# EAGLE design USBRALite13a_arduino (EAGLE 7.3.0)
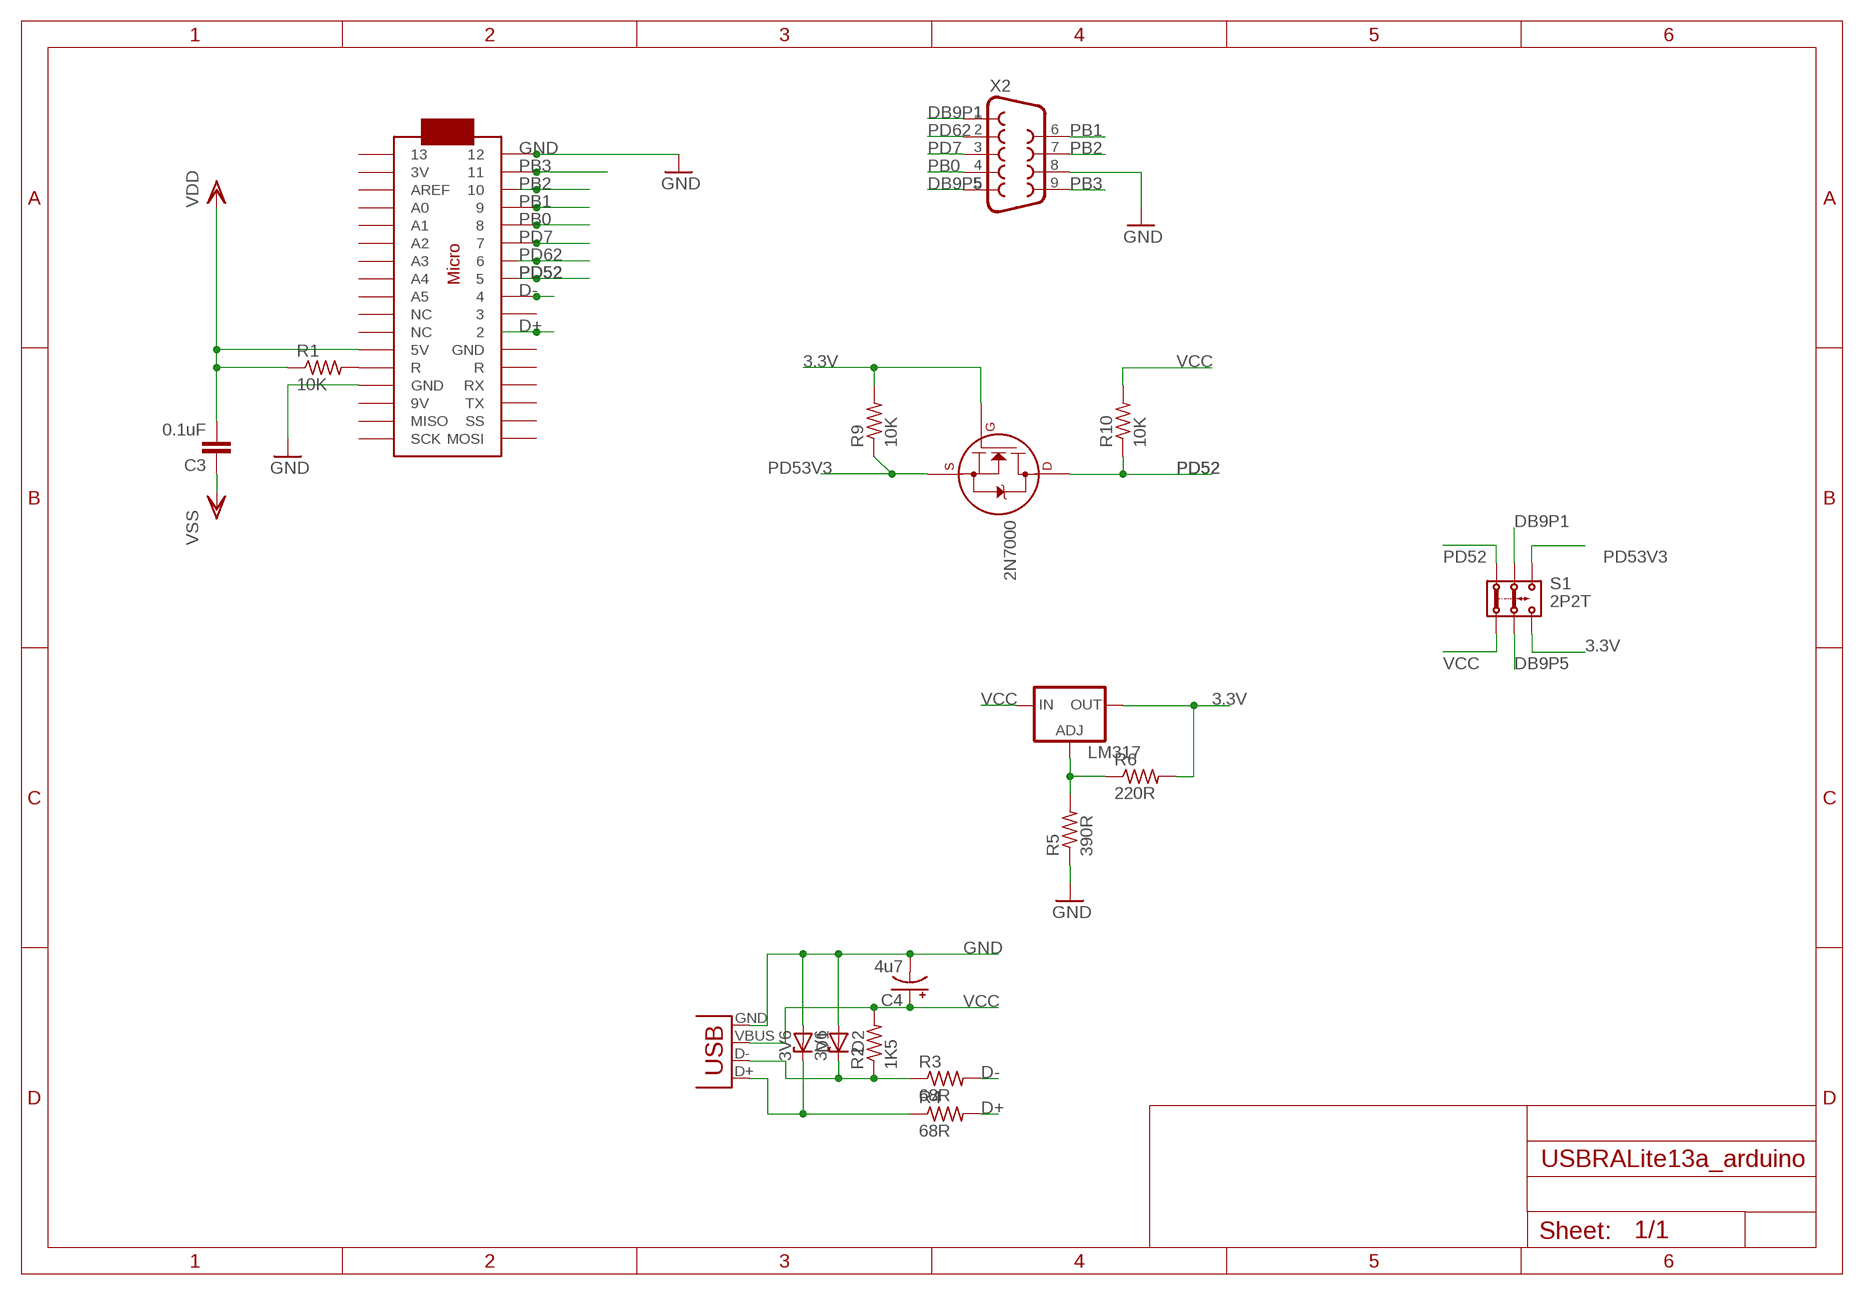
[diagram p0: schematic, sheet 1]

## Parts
2N7000  2N7000_TO92  [TO-92]
C3  0.1uF  C-EU050-024X044  [C050-024X044]
C4  4u7  CPOL-USE2.5-6  [E2,5-6]
D1  3V6  ZENER-DIODEZD-5  [ZDIO-5]
D2  3V6  ZENER-DIODEZD-5  [ZDIO-5]
LM317  LM317TS  [317TS]
R1  10K  R-US_0207/10  [0207/10]
R2  1K5  R-US_0207/10  [0207/10]
R3  68R  R-US_0207/10  [0207/10]
R4  68R  R-US_0207/10  [0207/10]
R5  390R  R-US_0207/10  [0207/10]
R6  220R  R-US_0207/10  [0207/10]
R9  10K  R-US_0207/10  [0207/10]
R10  10K  R-US_0207/10  [0207/10]
S1  2P2T  [2P2T]
U$2  ARDUINOMICRO  [ARDUINOMICRO]
X1  USBPTH  [USB-B-PTH]
X2  DB9MALE  [DB9_MALE]

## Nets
3.3V: 2N7000.2(G) LM317.2(OUT) R6.2 R9.2 S1.3.2
D+: R4.2 U$2.P$11
D-: R3.2 U$2.P$9
DB9P1: S1.2.1 X2.1
DB9P5: S1.2.2 X2.5
GND: C3.1 C4.- D1.A D2.A R5.1 U$2.P$1 U$2.P$12(GND) X1.GND X2.8 ; supply symbol labelled VSS
N$1: R1.2 U$2.P$13(R)
N$5: LM317.1(ADJ) R5.2 R6.1
N$8: D1.C R4.1 X1.D+
N$9: D2.C R2.1 R3.1 X1.D-
PB0: U$2.P$5 X2.4
PB1: U$2.P$4 X2.6
PB2: U$2.P$3 X2.7
PB3: U$2.P$2 X2.9
PD7: U$2.P$6 X2.3
PD52: 2N7000.3(D) R10.1 S1.1.1 U$2.P$8
PD53V3: 2N7000.1(S) R9.1 S1.3.1
PD62: U$2.P$7 X2.2
VCC: C3.2 C4.+ LM317.3(IN) R1.1 R2.2 R10.2 S1.1.2 U$2.P$23(5V) X1.VBUS ; supply symbol labelled VDD
Unconnected: U$2.P$10 U$2.P$14(RX) U$2.P$15(TX) U$2.P$16(SS) U$2.P$17(MOSI) U$2.P$18(SCK) U$2.P$19(MISO) U$2.P$20(9V) U$2.P$21(GND) U$2.P$22(R) U$2.P$24(NC) U$2.P$25(NC) U$2.P$26(A5) U$2.P$27(A4) U$2.P$28(A3) U$2.P$29(A2) U$2.P$30(A1) U$2.P$31(A0) U$2.P$32(AREF) U$2.P$33(3V) U$2.P$34

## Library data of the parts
2N7000 = transistors:2N700*: 2N7000, 2N7002, NDS7002A N-channel enhancement mode MOSFET
C3 = rcl:C-EU: CAPACITOR, European symbol
C4 = adafruit:CPOL-US: POLARIZED CAPACITOR, American symbol
D1 D2 = diode:ZENER-DIODE: Z-Diode
LM317 = v-reg:LM317TS: VOLTAGE REGULATOR
R1-R6 R9 R10 = adafruit:R-US_: RESISTOR, American symbol
S1 = Itead_BP_110825:2P2T: BAS011
U$2 = adafruit:ARDUINOMICRO
X1 = SparkFun:USB: USB Connectors USB-B-PTH is fully proven SKU : PRT-00139 USB-miniB is fully proven SKU : PRT-00587 USB-A-PCB is untested. USB-A-H is throughly reviewed, but untested. Spark Fun Electronics SKU : PRT-00437 USB-B-SMT is throughly reviewed, but untested. Needs silkscreen touching up. USB-A-S has not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
X2 = SparkFun:DB9: DB9 Connector Standard DB9 (D-Sub 9) serial connector. Can be used for CAN bus as well as RS485 and RS232. Footprint production proven. Spark Fun Electronics SKU : PRT-00429

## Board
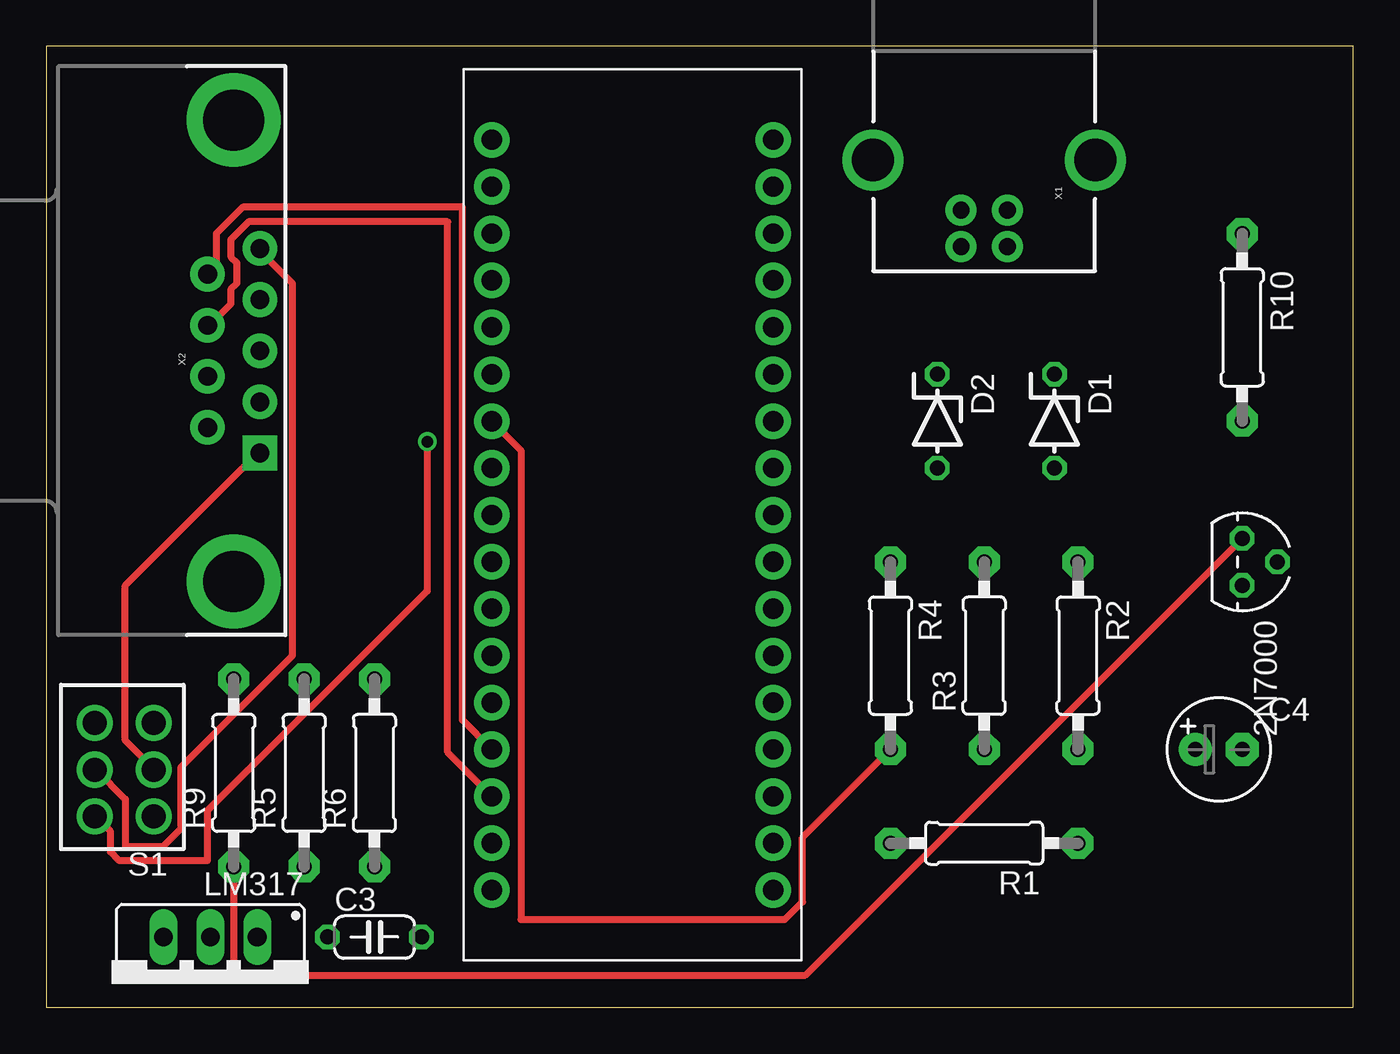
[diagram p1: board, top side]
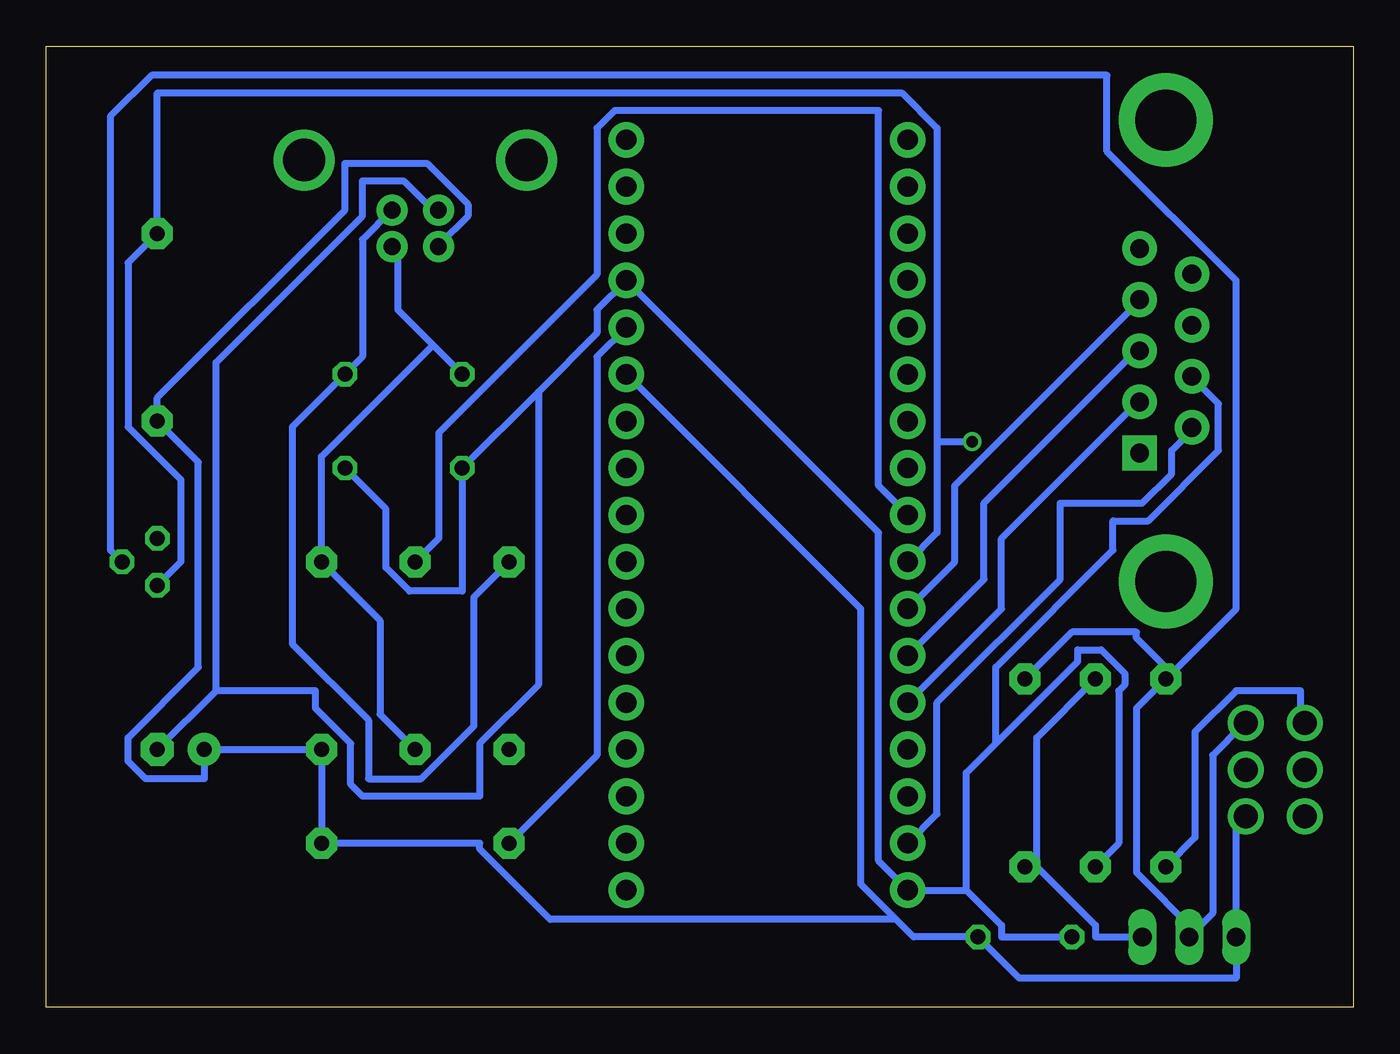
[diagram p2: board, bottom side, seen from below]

Size 70.79 x 52.06 mm. Coordinates in mm from the lower left corner, seen from the top.
Outline: 0,0 70.79,0 70.79,52.06 0,52.06 0,0
Copper layers (1*16): Top 0.035mm / dielectric 1.5mm / Bottom 0.035mm
Design rules "default *": minimum track width 15mil, minimum drill 24mil, track to track 12mil, track to pad 12mil, pad to pad 12mil, via to via 12mil, smd to smd 12mil, copper to edge 40mil, drill to drill 8mil, minimum pad ring 10mil, minimum via ring 8mil, stop-mask expansion 4mil, vias tented up to drill 0mil, thermal gap 10mil

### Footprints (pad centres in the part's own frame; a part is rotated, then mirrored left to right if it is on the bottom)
TO-92 = drill 0.813 octagon: 1 -1.27,0; 2 0,1.905; 3 1.27,0
C050-024X044 = drill 0.813 octagon: 1 -2.54,0; 2 2.54,0
E2,5-6 = drill 0.813 pad 1.778: + -1.27,0 | drill 0.813 pad 1.778 octagon: - 1.27,0
ZDIO-5 = drill 0.813 octagon: A 2.54,0; C -2.54,0
317TS = drill 1.016 long: 1 -2.54,-2.54; 2 0,-2.54; 3 2.54,-2.54
0207/10 = drill 0.813 pad 1.676 octagon: 1 -5.08,0; 2 5.08,0
2P2T = drill 1.3 pad 1.93: 1.1 -3.635,-0.085; 1.2 -3.635,-3.285; 2.1 -1.095,-0.085; 2.2 -1.095,-3.285; 3.1 1.445,-0.085; 3.2 1.445,-3.285
ARDUINOMICRO = drill 1.1 pad 1.93: P$1 -20.32,7.62; P$2 -17.78,7.62; P$3 -15.24,7.62; P$4 -12.7,7.62; P$5 -10.16,7.62; P$6 -7.62,7.62; P$7 -5.08,7.62; P$8 -2.54,7.62; P$9 0,7.62; P$10 2.54,7.62; P$11 5.08,7.62; P$12 12.7,-7.62; P$13 10.16,-7.62; P$14 12.7,7.62; P$15 15.24,7.62; P$16 17.78,7.62; P$17 20.32,7.62; P$18 20.32,-7.62; P$19 17.78,-7.62; P$20 15.24,-7.62; P$21 7.62,7.62; P$22 10.16,7.62; P$23 7.62,-7.62; P$24 5.08,-7.62; P$25 2.54,-7.62; P$26 0,-7.62; P$27 -2.54,-7.62; P$28 -5.08,-7.62; P$29 -7.62,-7.62; P$30 -10.16,-7.62; P$31 -12.7,-7.62; P$32 -15.24,-7.62; P$33 -17.78,-7.62; P$34 -20.32,-7.62
USB-B-PTH = drill 0.914 pad 1.676: D+ 0,1.25; D- 1.981,1.25; GND 0,-1.25; VBUS 1.981,-1.25 | drill 2.286: S1 -2.718,-6.02; S2 -2.718,6.02
DB9_MALE = drill 1.016 pad 1.88: 1 5.54,-1.42; 2 2.77,-1.42; 3 0,-1.42; 4 -2.77,-1.42; 6 4.15,1.42; 7 1.38,1.42; 8 -1.38,1.42; 9 -4.15,1.42 | drill 1.016 pad 1.88 square: 5 -5.54,-1.42 | drill 3.302 pad 5.08: G1 -12.5,0; G2 12.5,0

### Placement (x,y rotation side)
2N7000  64.77,24.13 270 top
C3  17.78,3.81 0 top
C4  63.5,13.97 0 top
D1  54.61,31.75 270 top
D2  48.26,31.75 270 top
LM317  8.89,1.27 180 top
R1  50.8,8.89 180 top
R2  55.88,19.05 270 top
R3  50.8,19.05 90 top
R4  45.72,19.05 270 top
R5  13.97,12.7 90 top
R6  17.78,12.7 90 top
R9  10.16,12.7 90 top
R10  64.77,36.83 270 top
S1  2.54,13.97 90 top
U$2  31.75,26.67 90 top
X1  50.8,43.18 270 top
X2  10.16,35.56 90 top

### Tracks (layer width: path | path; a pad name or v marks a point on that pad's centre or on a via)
3.3V
  Bottom 0.381: 8.57,4.13 7.62,5.08 7.62,13.65 6.03,15.24 S1.3.2 | 2N7000.2 67.31,24.76 67.31,48.26 65.09,50.48 13.34,50.48 13.34,46.36 6.35,39.37 6.35,21.59 9.84,18.1 | R6.2 15.24,20.32 11.75,20.32 11.75,20 9.84,18.1 | 9.84,18.1 R9.2 11.75,16.19 11.75,7.3 8.57,4.13 | 8.57,4.13 LM317.2
D+
  Top 0.381: R4.2 40.96,9.21 40.96,5.71 40.01,4.76 25.72,4.76 25.72,30.16 U$2.P$11
D-
  Bottom 0.381: R3.2 49.53,25.4 49.53,31.11 40.96,39.69 40.96,47.62 40.01,48.58 25.72,48.58 25.72,28.26 U$2.P$9
DB9P1
  Top 0.381: X2.1 11.59,40.96 13.34,39.21 13.34,19.05 7.3,13.02 7.3,9.68 6.35,8.73 4.29,8.73 4.29,11.27 2.7,12.86 S1.2.1
DB9P5
  Top 0.381: X2.5 11.43,30 4.29,22.86 4.29,14.45 5.71,13.02 S1.2.2
GND
  Bottom 0.381: 61.59,17.14 61.59,34.92 53.66,42.86 53.66,44.77 51.44,44.77 49.85,43.18 X1.GND | C4.- 61.59,17.14 | 44.13,33.34 40.96,36.51 40.96,37.78 U$2.P$12 25.72,25.72 25.72,7.94 U$2.P$1 20.95,6.35 | 44.13,33.34 D2.A 48.26,22.54 51.12,22.54 52.39,23.81 52.39,26.99 D1.A | C3.1 19.05,3.81 19.05,4.44 20.95,6.35 | R5.1 12.7,8.89 12.7,17.14 12.38,17.46 12.38,18.1 13.65,19.37 14.92,19.37 14.92,18.73 19.37,14.29 | 19.37,14.29 20.95,12.7 20.95,6.35 | 19.37,14.29 19.37,18.41 13.02,24.76 13.02,26.35 11.11,26.35 7.3,30.16 7.3,32.7 8.57,33.97 X2.8 | 61.59,17.14 56.2,17.14 56.2,16.19 54.29,14.29 54.29,12.07 53.66,11.43 47.31,11.43 47.31,14.29 44.13,17.46 44.13,33.34
N$1
  Bottom 0.381: R1.2 40.96,13.65 40.96,35.24 U$2.P$13
N$5
  Bottom 0.381: LM317.1 13.97,3.81 13.97,4.44 17.14,7.62 | R5.2 17.14,14.61 17.14,7.62 | 17.14,7.62 R6.1
N$8
  Bottom 0.381: X1.D+ 52.07,43.18 53.66,41.59 53.66,35.24 D1.C 57.47,31.43 57.47,19.68 53.34,15.56 53.34,12.38 50.48,12.38 47.62,15.24 47.62,22.22 R4.1
N$9
  Bottom 0.381: 49.85,35.88 51.75,37.78 51.75,40.96 X1.D- | 49.85,35.88 D2.C | R3.1 52.7,15.87 52.7,20.96 R2.1 55.88,29.84 49.85,35.88
PB0
  Bottom 0.381: U$2.P$5 19.05,21.59 19.05,25.4 11.75,32.7 X2.4
PB1
  Top 0.381: U$2.P$4 22.54,15.56 22.54,43.34 10.64,43.34 9.21,41.91 9.21,40.16 8.89,39.85 X2.6
PB2
  Top 0.381: U$2.P$3 21.75,13.81 21.75,42.55 10.95,42.55 10,41.59 10,40.64 10.32,40.32 10.32,39.21 10,38.89 10,38.1 8.89,36.99 X2.7
PB3
  Bottom 0.381: U$2.P$2 22.54,10.48 22.54,16.51 15.88,23.18 15.88,27.3 11.43,27.3 9.84,28.89 9.84,30.16 8.89,31.11 X2.9
PD7
  Bottom 0.381: U$2.P$6 20,23.18 20,27.3 11.75,35.56 X2.3
PD52  (via drill 0.61)
  Top 0.381: v20.64,30.64 20.64,22.54 8.73,10.64 8.73,7.94 3.97,7.94 3.49,8.41 3.49,9.53 2.7,10.32 S1.1.1
  Bottom 0.381: 2N7000.3 63.5,24.13 63.5,28.57 66.36,31.43 66.36,40.32 R10.1 64.77,49.53 24.45,49.53 22.54,47.62 22.54,30.64 | U$2.P$8 22.54,25.72 22.54,30.64 | 22.54,30.64 v20.64,30.64
PD53V3
  Top 0.381: 2N7000.1 41.12,1.75 10.16,1.75 R9.1
  Bottom 0.381: R9.1 8.57,9.21 8.57,14.92 6.35,17.14 2.86,17.14 2.86,15.56 S1.3.1
PD62
  Bottom 0.381: U$2.P$7 21.59,24.13 21.59,28.26 11.75,38.1 X2.2
VCC
  Bottom 0.381: X1.VBUS 49.53,41.28 47.94,42.86 47.94,43.5 50.16,45.72 54.61,45.72 54.61,43.18 64.77,33.02 R10.2 62.55,29.53 62.55,18.41 66.36,14.61 66.36,13.33 65.41,12.38 62.23,12.38 C4.+ R2.2 R1.1 47.31,8.89 47.31,8.57 43.5,4.76 24.77,4.76 | U$2.P$23 26.67,21.59 26.67,6.67 24.77,4.76 | 24.77,4.76 23.81,3.81 C3.2 18.1,1.59 6.35,1.59 LM317.3 6.35,9.84 6.03,10.16 S1.1.2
